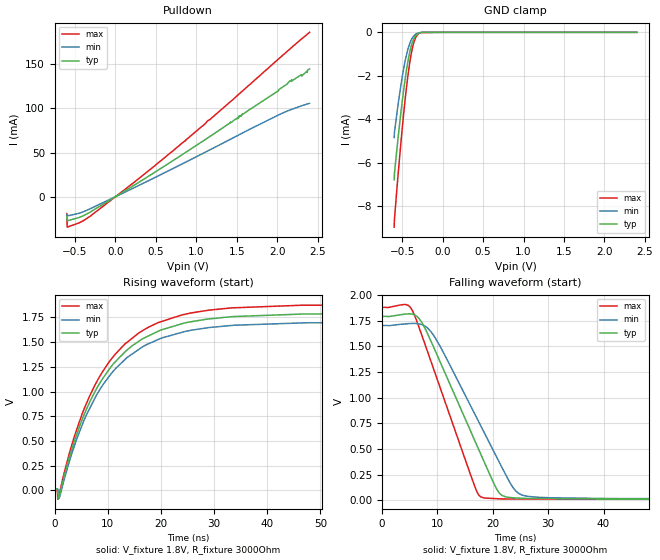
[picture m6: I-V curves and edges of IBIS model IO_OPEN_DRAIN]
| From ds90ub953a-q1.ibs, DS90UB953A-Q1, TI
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|   IO_OPEN_DRAIN Model
[Model]   IO_OPEN_DRAIN
Model_type   I/O_open_drain
Polarity   Non-Inverting
Enable   Active-Low
Vinl = 0.63
Vinh = 1.17
Vmeas = 0.9
Vref = 1.8
Cref = 2pF
Rref = 3000
|   typ   min   max
C_comp   0.6057pF   0.5862pF   0.6273pF
|C_comp_pull_down   0.2807pF   0.2159pF   0.3843pF
| Where Nom  PVT is Nominal Process, 1.8V, 27C
|   Fast PVT is Strong Process,  1.89V, -40C
|   Slow PVT is Weak Process,   1.71V, 105C
[Model spec]
|subparameter
Vinl   0.63   0.5985   0.6615
Vinh   1.17   1.1115   1.2285
[Voltage Range]   1.8   1.71   1.89
|Junction Temperature
[Temperature Range]   27   105   -40
[Pullup Reference]   1.8   1.71   1.89
[Pulldown Reference]   0   0   -0
[Power Clamp Reference]   1.8   1.71   1.89
[GND Clamp Reference]   0   0   0
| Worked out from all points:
|   slope of the pulldown table from 0 to 0.27 V, typ, clamps not added: 17.8 ohm
|   GND clamp passes 1 mA (typ) near -0.41 V on its own axis
|   falling waveform, V_fixture 1.8V, R_fixture 3000Ohm: 20-80 % time 8.72ns typ, 9.56ns min, 7.26ns max; typ from 1.79 V to 0.012 V
|   rising waveform, V_fixture 1.8V, R_fixture 3000Ohm: 20-80 % time 11ns typ, 11.1ns min, 11ns max; typ from 0.012 V to 1.79 V
[Pulldown]
|   Voltage   I(typ)   I(min)   I(max)
-600mV    -22.24mA   -20.12mA   -19.11mA
-597mV    -27.36mA   -21.79mA   -34.49mA
-322.5mV  -18mA      -14.1mA    -22.79mA
867mV     50.11mA    39.07mA    63.49mA
1.52V     88.72mA    69.72mA    115.6mA
1.528V    91.44mA    70.14mA    116.4mA
2.018V    121.2mA    92.65mA    156.1mA
2.175V    130.6mA    98.82mA    168.7mA
2.178V    132.5mA    98.92mA    168.9mA
2.372V    140.7mA    105mA      184.1mA
2.381V    143.7mA    105.2mA    184.7mA
2.4V      144.7mA    105.7mA    186.2mA
[GND Clamp]
|   Voltage   I(typ)   I(min)   I(max)
-600mV    -6.786mA   -4.845mA   -8.969mA
-597mV    -6.517mA   -4.622mA   -8.642mA
-595.5mV  -6.461mA   -4.578mA   -8.571mA
-553.5mV  -4.936mA   -3.381mA   -6.651mA
-517.5mV  -3.724mA   -2.457mA   -5.114mA
-477mV    -2.501mA   -1.563mA   -3.542mA
-432mV    -1.382mA   -805.2uA   -2.06mA
-402mV    -819.8uA   -460.4uA   -1.274mA
-367.5mV  -383.1uA   -214uA     -616.5uA
-333mV    -148.2uA   -86.87uA   -233uA
-294mV    -38.61uA   -24.56uA   -53.27uA
2.4V      0A         0A         0A
[POWER Clamp]
|   Voltage   I(typ)   I(min)   I(max)
-600mV    0A         0A         0A
0V        0A         0A         0A
2.4V      0A         0A         0A
[Ramp]
R_load = 3000
|   typ   min   max
dV/dt_r   1.06805/1.10257e-08   1.0134/1.10318e-08   1.12192/1.09287e-08
dV/dt_f   1.06846/8.72112e-09   1.01386/9.55589e-09   1.12226/7.25863e-09
[Falling Waveform]
V_fixture = 1.8V
V_fixture_min = 1.71V
V_fixture_max = 1.89V
R_fixture = 3000Ohm
C_fixture = 0F
|   Time   V(typ)   V(min)   V(max)
0s        1.792V     1.704V     1.88V
4.31ns    1.815V     1.72V      1.908V
5.611ns   1.812V     1.724V     1.835V
9.165ns   1.512V     1.619V     1.303V
16.88ns   566.3mV    827mV      117.1mV
18.25ns   398.2mV    681.4mV    25.65mV
21.53ns   53.58mV    333.6mV    14.1mV
24.58ns   22.12mV    71.09mV    12.98mV
27.81ns   17.92mV    31.23mV    11.79mV
147ns     11.73mV    14mV       9.992mV
[Rising Waveform]
V_fixture = 1.8V
V_fixture_min = 1.71V
V_fixture_max = 1.89V
R_fixture = 3000Ohm
C_fixture = 0F
|   Time   V(typ)   V(min)   V(max)
0s        11.73mV    14mV       9.992mV
427.2ps   11.51mV    13.57mV    9.631mV
601.8ps   -34.64mV   8.149mV    -90.06mV
845.8ps   -56.57mV   -79.68mV   -34.4mV
4.987ns   693.9mV    637.8mV    749.1mV
10.07ns   1.212V     1.142V     1.287V
15.96ns   1.514V     1.432V     1.597V
23.81ns   1.683V     1.597V     1.773V
47.02ns   1.784V     1.695V     1.872V
147ns     1.792V     1.703V     1.88V
